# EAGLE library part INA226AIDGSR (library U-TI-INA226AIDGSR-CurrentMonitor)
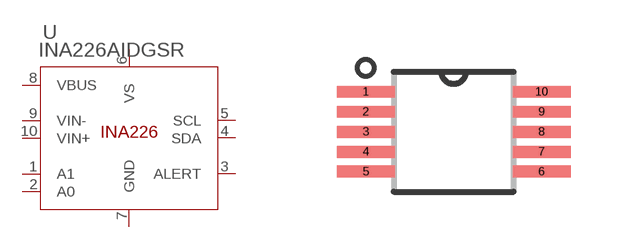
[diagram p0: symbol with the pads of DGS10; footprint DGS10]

Designator prefix U

## INA226AIDGSR (MANUFACTURER_PART_NUMBER: INA226AIDGSR; VENDOR: Texas Instruments)  [DGS10]
1  A1  pas
2  A0  pas
3  ALERT  out
4  SDA
5  SCL  in
6  VS  pwr
7  GND  pwr
8  VBUS  in
9  VIN-  in
10  VIN+  in

## Footprint DGS10 (pad centres in mm)
smd 1.45 x 0.3: 1 -2.2,1; 2 -2.2,0.5; 3 -2.2,0; 4 -2.2,-0.5; 5 -2.2,-1; 6 2.2,-1; 7 2.2,-0.5; 8 2.2,0; 9 2.2,0.5; 10 2.2,1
